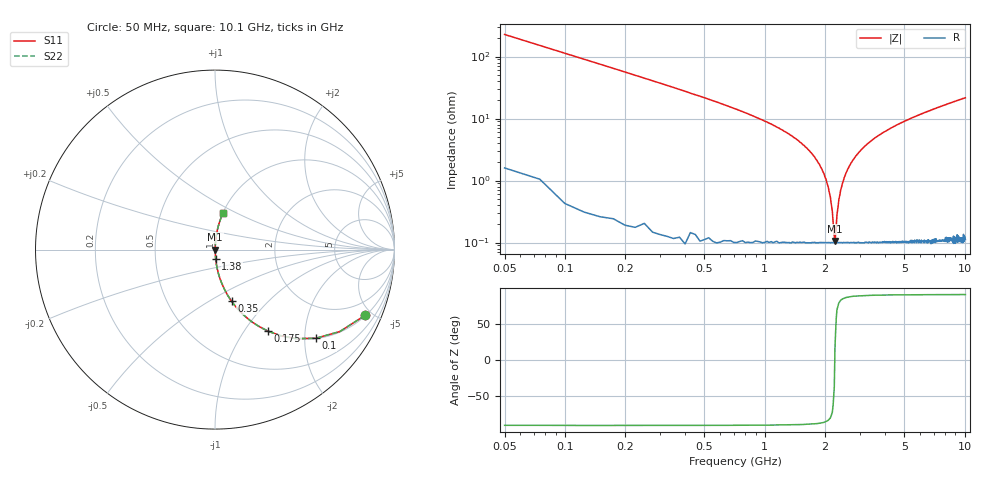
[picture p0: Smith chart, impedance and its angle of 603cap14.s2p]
! AVX Thin Film Operation		Date: November 2004
! Description: Accu-P® Series, Thin Film, SMD, RF Capacitor
! Part Number: 06033J140FBT
! 50 MHz  -  10.05 GHz
! Serial Measurements
# hz S db R 50
!	S11		S21		S12		S22
!	dB	Phase	dB	Phase	dB	Phase	dB	Phase
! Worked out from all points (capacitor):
!   400 points, 50 MHz to 10.1 GHz, reference 50 ohm
!   read as one part in series: C = 14 pF near 100 MHz
!   lowest |Z| = 106 mohm at 2.25 GHz (marker M1)
!   series resonance near 2.244 GHz, so ESL is about 360 pH
!   S11 on the Smith chart (normalised r, x): 50 MHz: 1.03, -4.54; 100 MHz: 1.01, -2.27; 175 MHz: 1.01, -1.29; 350 MHz: 1.00, -0.63; 1.38 GHz: 1.00, -0.10; 10.1 GHz: 1.00, +0.43
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5e7  -0.79 -23.7  -7.92 65.9  -7.92 65.9  -0.79 -23.7
1e8  -2.52 -41.3  -3.61 48.5  -3.61 48.5  -2.52 -41.3
1.75e8  -5.33 -57.0  -1.53 32.8  -1.53 32.8  -5.33 -57.0
3.5e8  -10.40 -72.2  -0.43 17.6  -0.43 17.6  -10.40 -72.2
7.25e8  -17.10 -81.6  -0.09 8.0  -0.09 8.0  -17.10 -81.6
1.38e9  -25.80 -85.9  -0.02 3.0  -0.02 3.0  -25.80 -85.9
1.73e9  -31.40 -86.3  -0.01 1.5  -0.01 1.5  -31.40 -86.3
1.93e9  -36.20 -85.4  -0.01 0.9  -0.01 0.9  -36.20 -85.4
2.08e9  -42.00 -82.3  -0.01 0.4  -0.01 0.4  -42.00 -82.3
2.18e9  -49.80 -71.8  -0.01 0.2  -0.01 0.2  -49.80 -71.8
2.23e9  -58.00 -37.4  -0.01 0.0  -0.01 0.0  -58.00 -37.4
2.25e9  -59.50 20.2  -0.01 -0.0  -0.01 -0.0  -59.50 20.2
2.3e9  -51.10 68.8  -0.01 -0.1  -0.01 -0.1  -51.10 68.8
2.35e9  -46.20 77.9  -0.01 -0.3  -0.01 -0.3  -46.20 77.9
2.45e9  -40.90 83.2  -0.01 -0.5  -0.01 -0.5  -40.90 83.2
2.55e9  -37.60 84.9  -0.01 -0.8  -0.01 -0.8  -37.60 84.9
2.85e9  -32.20 86.3  -0.01 -1.4  -0.01 -1.4  -32.20 86.3
3.4e9  -27.30 86.2  -0.02 -2.5  -0.02 -2.5  -27.30 86.2
5.08e9  -20.70 84.1  -0.05 -5.3  -0.05 -5.3  -20.70 84.1
6.75e9  -17.40 81.8  -0.09 -7.7  -0.09 -7.7  -17.40 81.8
8.43e9  -15.20 79.6  -0.14 -10.0  -0.14 -10.0  -15.20 79.6
1.01e10  -13.50 77.5  -0.21 -12.2  -0.21 -12.2  -13.50 77.5
